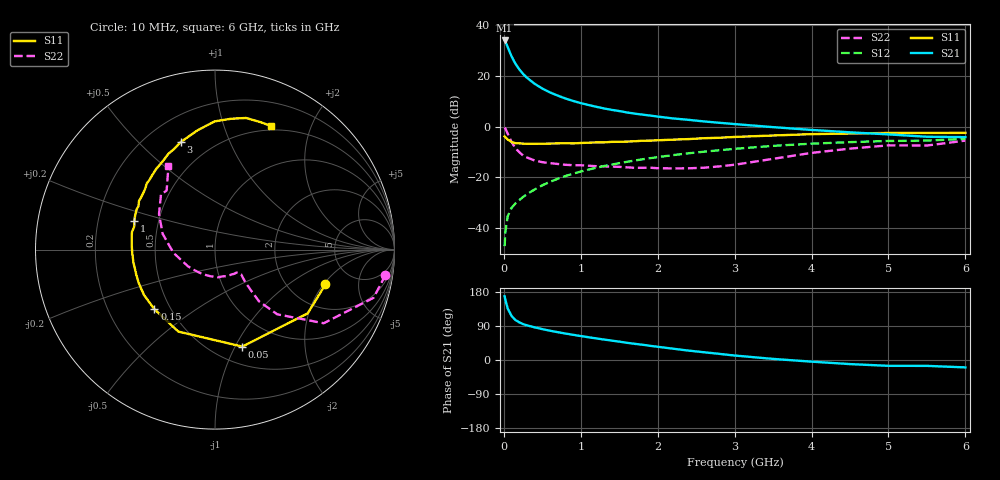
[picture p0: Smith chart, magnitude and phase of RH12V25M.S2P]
! SIEMENS Small Signal Semiconductors
! BFR106
! Si NPN RF Bipolar Junction Transistor in SOT23
! VCE = 12 V  IC = 25 mA
! Common Emitter S-Parameters:  August  1996
# GHz  S  MA  R  50
!  f  S11  S21  S12  S22
! GHz  MAG  ANG  MAG  ANG  MAG  ANG  MAG  ANG
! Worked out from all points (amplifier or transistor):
!   36 points, 10 MHz to 6 GHz, reference 50 ohm
!   highest |S21| = 34.0 dB at 10 MHz (marker M1)
!   |S21| within 3 dB of that: start of sweep to 55.32 MHz
!   unconditionally stable (mu >= 1): 360 MHz to 2.15 GHz
!   at 250 MHz: K = 0.90, MSG = 24.3 dB, |S12| = -27.7 dB
!   at 1.4 GHz: K = 1.06, MAG = 9.3 dB, |S12| = -14.9 dB
!   at 6 GHz: K = 0.98, MSG = 0.3 dB, |S12| = -4.8 dB
!   S11 on the Smith chart (normalised r, x): 10 MHz: 3.14, -2.09; 50 MHz: 0.68, -1.07; 150 MHz: 0.41, -0.35; 1 GHz: 0.36, +0.15; 3 GHz: 0.34, +0.67; 6 GHz: 0.45, +1.45
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0.01  0.6452 -17.5  50.38 168.2  0.0044 82.7  0.9604 -8.5
0.02  0.6269 -34.5  48.06 158.8  0.0084 74.7  0.9233 -16.9
0.05  0.5612 -74.3  37.28 136.0  0.0171 62.5  0.7317 -34.1
0.1  0.5004 -114.1  24.57 116.3  0.025 55.7  0.5005 -46.1
0.15  0.4735 -135.5  17.55 105.5  0.0306 55.5  0.379 -49.6
0.2  0.4696 -147.4  13.64 99.5  0.0357 58.3  0.3152 -48.8
0.25  0.464 -156.3  11.03 94.7  0.0411 60.1  0.2716 -47.8
0.3  0.4604 -162.4  9.268 91.5  0.0467 62.5  0.2475 -47.1
0.4  0.4601 -171.2  7.05 86.2  0.0578 65.1  0.2158 -44.8
0.5  0.4617 -178.2  5.664 81.5  0.0699 66.6  0.1997 -43.3
0.6  0.4651 176.3  4.759 77.3  0.0818 67.3  0.1915 -43.9
0.8  0.4728 168.1  3.608 69.9  0.1064 67.0  0.1775 -46.2
1  0.4776 160.2  2.927 63.2  0.1304 66.3  0.1737 -49.9
1.1  0.4845 156.6  2.684 60.1  0.1426 65.7  0.1701 -53.2
1.3  0.4905 150.4  2.299 54.0  0.1674 63.9  0.1649 -58.7
1.6  0.5096 141.6  1.914 45.4  0.2034 60.9  0.158 -70.2
2.2  0.5561 126.1  1.459 29.9  0.2755 53.7  0.1506 -99.3
3  0.6287 107.7  1.128 11.8  0.3662 42.9  0.1778 -149.1
3.5  0.6715 98.4  0.982 2.9  0.4195 35.6  0.2327 -175.7
4.5  0.7348 82.9  0.775 -10.8  0.4966 20.4  0.3699 147.5
5.5  0.754 70.3  0.634 -15.5  0.5331 9.5  0.4255 129.3
6  0.7561 65.8  0.624 -19.5  0.5768 2.1  0.5329 119.1
